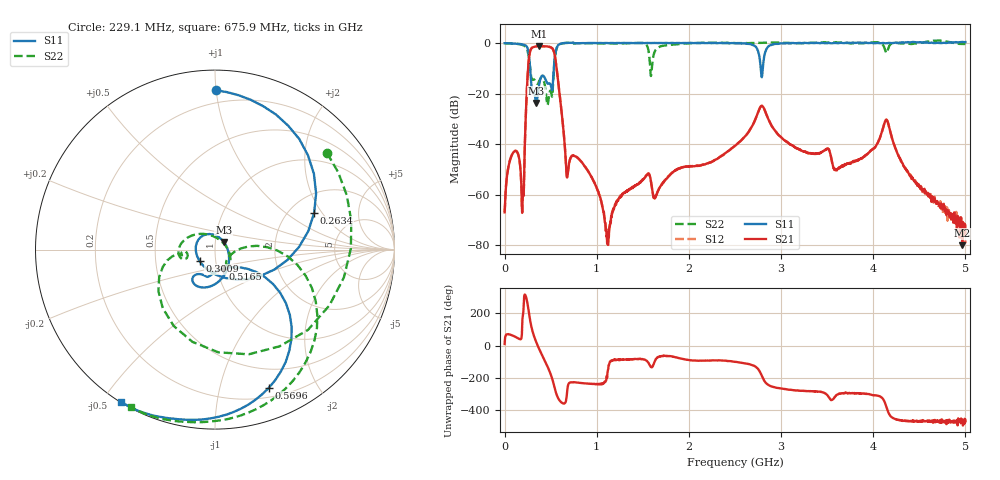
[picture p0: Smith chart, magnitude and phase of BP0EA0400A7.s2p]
!Agilent Technologies,E8358A,US41080443,A.07.50.56
!Agilent E8358A: A.07.50.56
!Date: Friday, November 10, 2017 09:15:52
!Correction: S11(Full 2 Port(1,2))
!S21(Full 2 Port(1,2))
!S12(Full 2 Port(1,2))
!S22(Full 2 Port(1,2))
!S2P File: Measurements: S11, S21, S12, S22:
# Hz S  dB  R 50
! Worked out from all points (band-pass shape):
!   1601 points, 1 MHz to 5 GHz, reference 50 ohm
!   highest |S21| = -1.30 dB at 375.9 MHz (marker M1); lowest = -79.9 dB at 4.966 GHz (marker M2)
!   |S21| within 3 dB of the highest: 272.1 MHz to 541.4 MHz (269.3 MHz wide, 66.2 % of centre)
!   lowest |S11| = -23.7 dB at 344.7 MHz (marker M3), VSWR 1.14, Z = 54.9 + j4.76 ohm
!   |S11| at or under -10 dB: 277.8 MHz to 535.2 MHz (257.4 MHz wide, 63.3 % of centre); 2.78 GHz to 2.802 GHz (22.45 MHz wide, 0.805 % of centre)
!   |S22| runs from -24.7 to 0.9 dB; largest |S21 - S12| = 0.0046
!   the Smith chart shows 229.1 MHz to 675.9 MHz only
!   S11 on the Smith chart (normalised r, x): 229.1 MHz: 0.12, +1.00; 263.4 MHz: 2.70, +1.69; 300.9 MHz: 0.84, -0.11; 516.5 MHz: 1.07, -0.23; 569.6 MHz: 0.29, -1.42; 675.9 MHz: 0.00, -0.56
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1000000  -0.14 179.8  -66.93 10.5  -66.78 11.3  -0.16 179.8
1.0098e8  -0.27 157.0  -43.04 59.2  -42.98 59.8  -0.30 152.0
1.947112e8  -0.61 119.9  -64.01 168.8  -63.08 170.0  -0.83 98.9
2.290794e8  -1.04 89.8  -30.36 -51.4  -30.30 -51.4  -1.68 40.7
2.634475e8  -4.60 20.3  -6.68 -151.2  -6.63 -151.2  -5.53 -103.7
3.0094e8  -19.41 -143.4  -1.90 95.8  -1.85 95.7  -14.60 -170.5
3.446812e8  -23.73 41.5  -1.38 21.3  -1.34 21.3  -15.89 -174.8
3.75925e8  -16.33 -70.8  -1.30 -20.3  -1.26 -20.2  -15.06 -162.3
4.446612e8  -14.47 -128.8  -1.36 -101.2  -1.33 -101.2  -18.50 132.4
5.165219e8  -18.71 -67.9  -2.12 157.3  -2.09 157.3  -21.27 -31.2
5.696362e8  -1.65 -68.8  -11.42 51.2  -11.39 51.2  -1.86 -51.4
6.75865e8  -0.02 -121.6  -52.90 57.7  -52.81 57.8  -0.04 -118.1
8.352081e8  -0.11 -144.0  -47.05 129.1  -46.99 128.9  -0.13 -141.8
1.119526e9  -0.09 -160.1  -78.99 -157.4  -79.30 -161.4  -0.23 -167.5
1.669416e9  -0.07 -172.8  -58.20 -68.3  -58.17 -68.5  -1.81 -115.4
2.5005e9  -0.19 168.7  -40.69 -99.4  -40.63 -99.4  -0.10 -179.4
2.787942e9  -13.16 16.8  -24.89 178.2  -24.86 178.7  0.03 174.9
2.916042e9  -0.58 -162.2  -33.75 105.3  -33.74 105.4  0.12 179.0
3.334708e9  -0.03 172.9  -43.70 78.6  -43.75 78.4  0.04 164.6
4.168916e9  -0.01 156.0  -32.71 -58.6  -32.73 -57.9  -1.63 177.4
4.965632e9  0.38 143.8  -79.91 -115.4  -73.71 -102.2  -0.41 151.7
5e9  0.30 144.3  -74.79 -106.9  -79.12 -130.0  -0.48 151.1
